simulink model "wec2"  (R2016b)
settings: Solver=ode4  StartTime=0  StopTime=350  FixedStep=0.005  MaxStep=0.005  RelTol=1e-3  EnableMultiTasking=on
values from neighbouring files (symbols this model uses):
  arAdaptiveLawData = 1/2*zModelSimple.zModelPto.arFreq.*     zModelSimple.zModelPto.arMagnitude./     cos(zModelSimple.zModelPto.arPhase*pi/180+pi/2)    [IMPACT_Control.m]
  arControllerRampGain = [0,0,1,1]    [IMPACT_Control.m]
  arControllerRampTime = [0 rStartRampTime rStartRampTime+rRampTimeLength 8000]    [IMPACT_Control.m]
  arEkfInitialisation = zeros(1,11)    [IMPACT_Control.m]
  arFrequency = zModelSimple.zModelPto.arFreq    [IMPACT_Control.m]
  arFrequencyRange = zModelSimple.zModelPto.arFreq    [IMPACT_Control.m]
  arImpedance = 1./zModelSimple.zModelPto.arMagnitude./zModelSimple.zModelPto.arFreq    [IMPACT_Control.m]
  iAdaptiveDamping = 0    [wec2_IMPACT_Project.m]    (also in IMPACT_Control.m = handles.iAdaptiveDamping; wec1_IMPACT_Project.m; wec3_IMPACT_Project.m; wec4IMPACT_Project.m)
  iControlType = 1    [wec2_IMPACT_Project.m]    (also in IMPACT_Control.m = handles.iControlType; wec1_IMPACT_Project.m; wec3_IMPACT_Project.m; wec4IMPACT_Project.m = 2)
  iPtoPositionConstraint = 1    [wec2_IMPACT_Project.m]    (also in IMPACT_Control.m = handles.iPtoPositionConstraint; wec1_IMPACT_Project.m = 0; wec3_IMPACT_Project.m; wec4IMPACT_Project.m)
  iSensorNoise = 0    [IMPACT_Control.m]
  m = m+1    (= 2)    [checkParamFile.m]
  rAccelerationGainPosLim = 4.5133e+06    (= 4513300)    [wec2AdditionalParams.m]    (also in wec1AdditionalParams.m = 9453000)
  rBalancingForce = -(rFloaterVolume*rDENSITY - rFloaterMass)*rGRAVITY    [IMPACT_Control.m]
  rBuoyancyGainPosLim = 7.4216    [wec2AdditionalParams.m]    (also in wec1AdditionalParams.m = 3135500)
  rCogFloater = -8.5    [wec2_IMPACT_Model.m]    (also in paramInitial.m = get( handles.edit_rCogFloater, 'String' ); wec1_IMPACT_Model.m = -18; wec3_IMPACT_Model.m = -0.7; wec3_IMPACT_Model2.m = -0.7)
  rDampingGainPosLim = 1.1575e+04    (= 11575)    [wec2AdditionalParams.m]    (also in wec1AdditionalParams.m = 203690)
  rDisplacementLimit = 10.000000    (= 10)    [wec2_IMPACT_Project.m]    (also in IMPACT_Control.m = getValue(handles.edit_displacementLimit); wec1_IMPACT_Project.m; wec3_IMPACT_Project.m = 3; wec4IMPACT_Project.m)
  rGainForAntiWIndUp = tfControllerDiscrete.rGain    [IMPACT_Control.m]
  rMaxForcePto = 1000000000000000.000000    (= 1e+15)    [wec2_IMPACT_Project.m]    (also in IMPACT_Control.m = getValue(handles.edit_maxForcePto); wec1_IMPACT_Project.m; wec3_IMPACT_Project.m = 1000000000; wec4IMPACT_Project.m = 300000000)
  rMinForcePto = -1000000000000000.000000    (= -1e+15)    [wec2_IMPACT_Project.m]    (also in IMPACT_Control.m = getValue(handles.edit_minForcePto); wec1_IMPACT_Project.m; wec3_IMPACT_Project.m = -1000000000; wec4IMPACT_Project.m = -300000000)
  rOutputSampleTime = 0.010000    (= 0.01)    [wec2_IMPACT_Project.m]    (also in IMPACT_Control.m = getValue(handles.edit_outputSampleTime); wec1_IMPACT_Project.m; wec3_IMPACT_Project.m; wec4IMPACT_Project.m)
  rPassiveDampingGain = -1948070.000000    (= -1948070)    [wec2_IMPACT_Project.m]    (also in IMPACT_Control.m = getValue(handles.edit_gainPLD); wec1_IMPACT_Project.m = -214018.1537; wec3_IMPACT_Project.m = -519390; wec4IMPACT_Project.m = -604830)
  rPositionLimitRatio = 10    [wec2AdditionalParams.m]    (also in wec1AdditionalParams.m)
  rUpperFrequencyLimit = EKFFloater.upperFreq    [IMPACT_Control.m]
  s = tf('s')    [wec2_IMPACT_Model.m]    (also in IMPACT_Control.m; wec1_IMPACT_Model.m; wec3_IMPACT_Model.m; wec3_IMPACT_Model2.m)
  simu = simulationClass()    [wecSimInputFile.m]
  Z = magPhaseToComplex(zModelTf)    [IMPACT_Control.m]
undefined symbols (not defined in the file or in its folder): arControllerDiscreteDen, arControllerDiscreteNum, arExcForceFloaterDen, arExcForceFloaterNum, body, N, pto, rAccelerationGainFloater, rBuoyancyGainFloater, rDampingGainFloater, X, Y
libraries: nesl_utility x9, sm_lib x5, simulink x3, WECSim_Lib x2

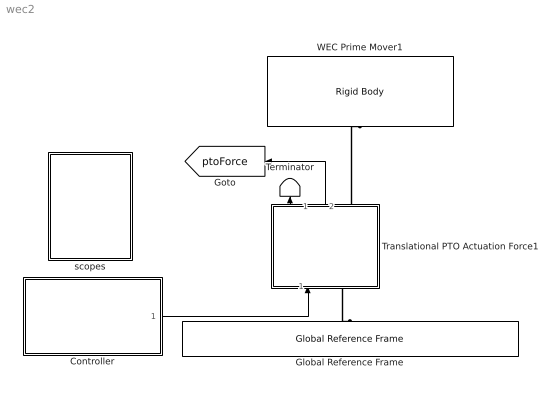
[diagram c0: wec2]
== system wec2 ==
  Controller : Subsystem
  Global Reference Frame : WECSim_Lib/Frames/Global Reference Frame  waves=waves  simu=simu
  Terminator : Terminator
  Translational PTO Actuation Force1 : Subsystem  AncestorBlock=WECSim_Lib/PTOs/Translational PTO Actuation Force
  WEC Prime Mover1 : WECSim_Lib/Body Elements/Rigid Body  body=body(1)
  scopes : Subsystem
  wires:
  Translational PTO Actuation Force1/2(ptoForce) -> [ptoForce]
  Controller/1(forceDemand) -> Translational PTO Actuation Force1/1(Force)
  Translational PTO Actuation Force1/1(Response) -> Terminator/1
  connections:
  Translational PTO Actuation Force1/LConn1 -- Global Reference Frame/RConn1
  Translational PTO Actuation Force1/RConn1 -- WEC Prime Mover1/RConn1

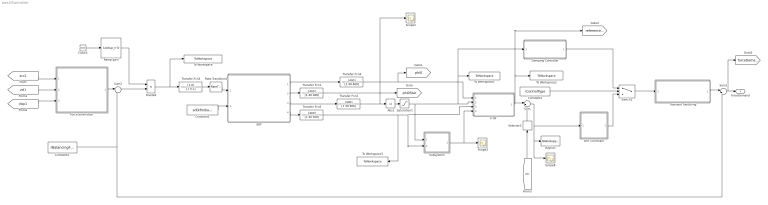
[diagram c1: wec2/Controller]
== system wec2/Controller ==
  Abs1 : Abs
  Clock3 : Clock
  Constant1 : Constant  Value=arEkfInitialisation
  Constant2 : Constant  Value=iControlType
  Constant5 : Constant  Value=rBalancingForce
  Damping Controller : Subsystem
  Divide4 : Product  Inputs=**
  EKF : MATLAB Function  TreatAsAtomicUnit=on
  "Force estimation " : Subsystem
  OVT Controller : Subsystem
  Ramp gain : Lookup_n-D  NumberOfTableDimensions=1  BreakpointsForDimension1=[0 5 10 8000]  Table=[0 0 1 1]  InternalRulePriority=Speed  RndMeth=Simplest
  Rate Transition1 : RateTransition  OutPortSampleTimeMultiple=0.01  OutPortSampleTime=0.01
  Saturation1 : Saturate  UpperLimit=rUpperFrequencyLimit  LowerLimit=0  LinearizeAsGain=off
  Scope2 : Scope
  Scope3 : Scope
  Scope8 : Scope
  Selector2 : Selector  InputPortWidth=6  IndexOptions=Index vector (dialog)  Indices=3  OutputSizes=1
  Subsystem : Subsystem
  Sum : Sum  Inputs=|+-
  Sum1 : Sum  Inputs=|++
  Sum2 : Sum  Inputs=|++
  Switch1 : Switch  Threshold=2
  To Workspace : ToWorkspace  VariableName=arEstimatedExcitationForce  SampleTime=rOutputSampleTime
  To Workspace1 : ToWorkspace  VariableName=arEkfFrequency  SampleTime=rOutputSampleTime
  To Workspace2 : ToWorkspace  VariableName=arReferenceVelocity  SampleTime=rOutputSampleTime
  To Workspace3 : ToWorkspace  VariableName=arEkfAmplitude  SampleTime=rOutputSampleTime
  Transfer Fcn{1..2,4..5} (4 alike) : TransferFcn  Numerator=[400]  Denominator=[1 40 400]
  Transfer Fcn3 : TransferFcn  Numerator=[1 0]  Denominator=[1 0.1]
  Transient Switching : Subsystem
  "V ref " : Subsystem
  output1 : ToWorkspace  VariableName=arError  SampleTime=rOutputSampleTime
  forceDemand : Outport
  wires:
  Damping Controller/1(forceDemand) -> Switch1/1
  Sum/1 -> output1/1, Scope8/1, OVT Controller/1(error)
  Selector2/1 -> Sum/2
  "V ref "/1(referenceVelocity) -> Sum/1, To Workspace2/1, [referenceVelocity]
  [vel1] -> Selector2/1
  Constant2/1 -> Switch1/2
  OVT Controller/1(forceDemand) -> Switch1/3
  Saturation1/1 -> Subsystem/1(frequency), Damping Controller/1(ekfFrequency), To Workspace1/1, "V ref "/2(ekfFrequency)
  [acc1] -> "Force estimation "/1(Acceleration)
  [vel1] -> "Force estimation "/2(Velocity)
  [disp1] -> "Force estimation "/3(Position)
  Abs1/1 -> Saturation1/1
  "Force estimation "/1(estimatedExcitationForce) -> Sum2/1
  Sum1/1 -> [forceDemand], forceDemand/1
  Constant1/1 -> EKF/2(arEkfInitialisation)
  Constant5/1 -> Sum1/2, Sum2/2
  Switch1/1 -> Transient Switching/1(forceDemandIn)
  Transient Switching/1(forceDemandOut) -> Sum1/1
  Rate Transition1/1 -> EKF/1(rEstimatedExcitationForce)
  Sum2/1 -> Divide4/2
  EKF/4(rAmplitudeOutput) -> Transfer Fcn5/1
  EKF/3(rFrequencyOutput) -> Transfer Fcn2/1
  EKF/1(rPhi0Output) -> Transfer Fcn4/1
  EKF/2(rPhi0StarOutput) -> Transfer Fcn1/1
  Transfer Fcn5/1 -> Subsystem/2(excitationForce), "V ref "/3(ekfAmplitude), To Workspace3/1
  Transfer Fcn2/1 -> Abs1/1, Scope2/1
  Transfer Fcn1/1 -> [phi0Star]
  Transfer Fcn4/1 -> [phi0], "V ref "/1(phiOut)
  Subsystem/1(displacementLimit) -> Scope3/1, "V ref "/4(displacementLimit)
  Clock3/1 -> Ramp gain/1
  Ramp gain/1 -> Divide4/1
  Divide4/1 -> To Workspace/1, Transfer Fcn3/1
  Transfer Fcn3/1 -> Rate Transition1/1

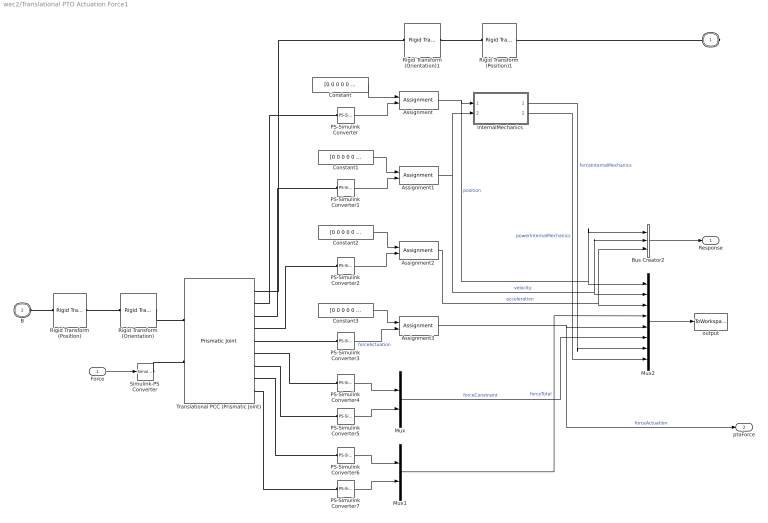
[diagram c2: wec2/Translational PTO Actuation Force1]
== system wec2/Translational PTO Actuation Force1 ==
  Force : Inport
  Assignment{,1..3} (4 alike) : Assignment  IndexOptions=Index vector (dialog)  Indices=3  OutputSizes=1
  Bus Creator2 : BusCreator  Inputs=3
  Constant{,1..3} (4 alike) : Constant  Value=[0 0 0 0 0 0]
  InternalMechanics : Subsystem
  Mux : Mux  Inputs=2
  Mux1 : Mux  Inputs=2
  Mux2 : Mux  Inputs=8
  PS-Simulink Converter{,1..7} (8 alike) : nesl_utility/PS-Simulink Converter  PhysicalDomain=network_engine_domain  SubClassName=ps_output  LeftPortType=input  RightPortType=output  PseudoPeriodic=off  Frequencies=[]  Unit=1  AffineConversion=off
  Rigid Transform (Position) : sm_lib/Frames and Transforms/Rigid Transform  TranslationMethod=Cartesian  TranslationStandardOffset=0  TranslationLengthUnit=m  TranslationStandardAxis=+Z  TranslationCartesianOffset=pto.initDisp.initLinDisp + pto.loc  TranslationROffset=0  TranslationROffsetUnits=m  TranslationZOffset=0  TranslationZOffsetUnits=m  TranslationThetaOffset=0  TranslationThetaOffsetUnits=deg  RotationMethod=None  RotationAngleUnits=rad  RotationStandardAxis=+Y  RotationAngle=0  RotationArbitraryAxis=[0 1 0]  FollAlignAxisA=+X  BaseAlignAxisA=+Y  FollAlignAxisB=+Y  BaseAlignAxisB=+Z  RotationSequenceAxes=FollowerAxes  RotationSequence=XYX  RotationSequenceAngles=[0 0 0]  RotationSequenceAnglesUnits=deg  RotationMatrix=[1 0 0; 0 1 0; 0 0 1]
  Rigid Transform (Position)1 : sm_lib/Frames and Transforms/Rigid Transform  TranslationMethod=Cartesian  TranslationStandardOffset=0  TranslationLengthUnit=m  TranslationStandardAxis=+Z  TranslationCartesianOffset=pto.initDisp.initLinDisp + pto.loc  TranslationROffset=0  TranslationROffsetUnits=m  TranslationZOffset=0  TranslationZOffsetUnits=m  TranslationThetaOffset=0  TranslationThetaOffsetUnits=deg  RotationMethod=None  RotationAngleUnits=rad  RotationStandardAxis=+Y  RotationAngle=0  RotationArbitraryAxis=[0 1 0]  FollAlignAxisA=+X  BaseAlignAxisA=+Y  FollAlignAxisB=+Y  BaseAlignAxisB=+Z  RotationSequenceAxes=FollowerAxes  RotationSequence=XYX  RotationSequenceAngles=[0 0 0]  RotationSequenceAnglesUnits=deg  RotationMatrix=[1 0 0; 0 1 0; 0 0 1]
  Rigid Transform (Orientation) : sm_lib/Frames and Transforms/Rigid Transform  TranslationMethod=None  TranslationStandardOffset=0  TranslationLengthUnit=m  TranslationStandardAxis=+Z  TranslationCartesianOffset=0  TranslationROffset=0  TranslationROffsetUnits=m  TranslationZOffset=0  TranslationZOffsetUnits=m  TranslationThetaOffset=0  TranslationThetaOffsetUnits=deg  RotationMethod=RotationMatrix  RotationAngleUnits=rad  RotationStandardAxis=+Y  RotationAngle=0  RotationArbitraryAxis=[0 1 0]  FollAlignAxisA=+X  BaseAlignAxisA=+Y  FollAlignAxisB=+Y  BaseAlignAxisB=+Z  RotationSequenceAxes=FollowerAxes  RotationSequence=XYX  RotationSequenceAngles=[0 0 0]  RotationSequenceAnglesUnits=deg  RotationMatrix=pto.orientation.rotationMatrix
  Rigid Transform (Orientation)1 : sm_lib/Frames and Transforms/Rigid Transform  TranslationMethod=None  TranslationStandardOffset=0  TranslationLengthUnit=m  TranslationStandardAxis=+Z  TranslationCartesianOffset=0  TranslationROffset=0  TranslationROffsetUnits=m  TranslationZOffset=0  TranslationZOffsetUnits=m  TranslationThetaOffset=0  TranslationThetaOffsetUnits=deg  RotationMethod=RotationMatrix  RotationAngleUnits=rad  RotationStandardAxis=+Y  RotationAngle=0  RotationArbitraryAxis=[0 1 0]  FollAlignAxisA=+X  BaseAlignAxisA=+Y  FollAlignAxisB=+Y  BaseAlignAxisB=+Z  RotationSequenceAxes=FollowerAxes  RotationSequence=XYX  RotationSequenceAngles=[0 0 0]  RotationSequenceAnglesUnits=deg  RotationMatrix=pto.orientation.rotationMatrix
  Simulink-PS Converter : nesl_utility/Simulink-PS Converter  PhysicalDomain=network_engine_domain  SubClassName=ps_input  LeftPortType=input  RightPortType=output  PseudoPeriodic=off  Frequencies=[]  NoiseDistribution=none  NoiseParameters=[]  Unit=1  AffineConversion=off  InputFiltering=off  SimscapeFilterOrder=1  InputFilterTimeConstant=0.001  UdotUserProvided=1
  Translational PCC (Prismatic Joint) : sm_lib/Joints/Prismatic Joint  SenseConstraintForce=on  SenseConstraintForceX=off  SenseConstraintForceY=off  SenseConstraintForceZ=off  SenseConstraintTorque=on  SenseConstraintTorqueX=off  SenseConstraintTorqueY=off  SenseConstraintTorqueZ=off  SenseTotalForce=on  SenseTotalForceX=off  SenseTotalForceY=off  SenseTotalForceZ=off  SenseTotalTorque=on  SenseTotalTorqueX=off  SenseTotalTorqueY=off  SenseTotalTorqueZ=off  CompositeWrenchDir=BaseOnFollower  CompositeWrenchFrame=BaseFrame  EquilibriumPosition=0  EquilibriumPositionUnits=m  SpringStiffness=pto.k  SpringStiffnessUnits=N/m  DampingCoefficient=pto.c  DampingCoefficientUnits=N/(m/s)  TorqueActuationMode=InputTorque  MotionActuationMode=ComputedMotion  SensePosition=on  SenseVelocity=on  SenseAcceleration=on  SenseTorqueForce=on  PositionTargetSpecify=off  PositionTargetPriority=High  PositionTargetValue=0  PositionTargetValueUnits=m  VelocityTargetSpecify=off  VelocityTargetPriority=High  VelocityTargetValue=0  VelocityTargetValueUnits=m/s
  output : ToWorkspace  VariableName=pto1_out  SaveFormat=Structure With Time  SampleTime=-1
  F : PMIOPort  Port=1  Side=Right
  B : PMIOPort  Port=2  Side=Left
  Response : Outport
  ptoForce : Outport  Port=2
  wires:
  Bus Creator2/1 -> Response/1
  Assignment/1 -> Mux2/1, Bus Creator2/1, InternalMechanics/1(Position)  "position"
  Assignment1/1 -> Mux2/2, Bus Creator2/2, InternalMechanics/2(Velocity)  "velocity"
  Assignment2/1 -> Mux2/3, Bus Creator2/3  "acceleration"
  Force/1 -> Simulink-PS Converter/1
  Mux2/1 -> output/1
  Mux/1 -> Mux2/6  "forceConstraint"
  Mux1/1 -> Mux2/4  "forceTotal"
  PS-Simulink Converter4/1 -> Mux/1
  PS-Simulink Converter5/1 -> Mux/2
  PS-Simulink Converter6/1 -> Mux1/1
  PS-Simulink Converter7/1 -> Mux1/2
  Assignment3/1 -> ptoForce/1, Mux2/5  "forceActuation"
  Constant/1 -> Assignment/1
  PS-Simulink Converter/1 -> Assignment/2
  Constant1/1 -> Assignment1/1
  PS-Simulink Converter1/1 -> Assignment1/2
  Constant2/1 -> Assignment2/1
  PS-Simulink Converter2/1 -> Assignment2/2
  InternalMechanics/1(Force) -> Mux2/7  "forceInternalMechanics"
  InternalMechanics/2(Power) -> Mux2/8  "powerInternalMechanics"
  Constant3/1 -> Assignment3/1
  PS-Simulink Converter3/1 -> Assignment3/2  "forceActuation"
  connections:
  Rigid Transform (Position)/RConn1 -- Rigid Transform (Orientation)/LConn1
  Rigid Transform (Position)1/RConn1 -- Rigid Transform (Orientation)1/LConn1
  Simulink-PS Converter/RConn1 -- Translational PCC (Prismatic Joint)/LConn2
  Rigid Transform (Orientation)/RConn1 -- Translational PCC (Prismatic Joint)/LConn1
  Rigid Transform (Position)/LConn1 -- B/RConn1
  Translational PCC (Prismatic Joint)/RConn5 -- PS-Simulink Converter3/LConn1
  Translational PCC (Prismatic Joint)/RConn9 -- PS-Simulink Converter7/LConn1
  Rigid Transform (Orientation)1/RConn1 -- Translational PCC (Prismatic Joint)/RConn1
  Translational PCC (Prismatic Joint)/RConn4 -- PS-Simulink Converter2/LConn1
  Translational PCC (Prismatic Joint)/RConn7 -- PS-Simulink Converter5/LConn1
  Translational PCC (Prismatic Joint)/RConn3 -- PS-Simulink Converter1/LConn1
  Rigid Transform (Position)1/LConn1 -- F/RConn1
  Translational PCC (Prismatic Joint)/RConn8 -- PS-Simulink Converter6/LConn1
  Translational PCC (Prismatic Joint)/RConn2 -- PS-Simulink Converter/LConn1
  Translational PCC (Prismatic Joint)/RConn6 -- PS-Simulink Converter4/LConn1

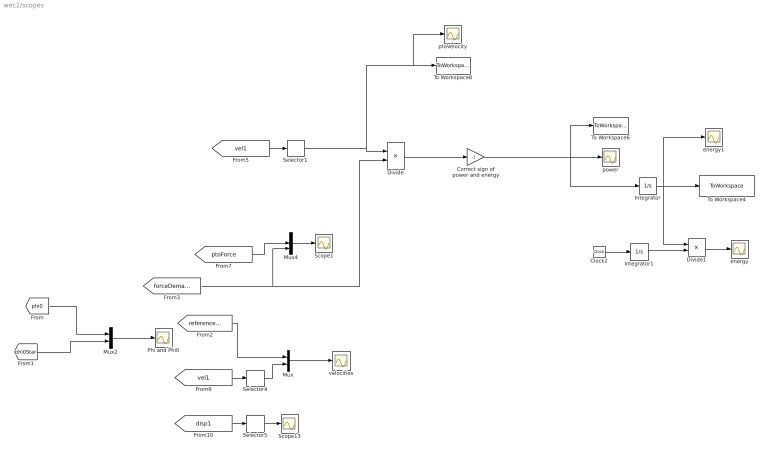
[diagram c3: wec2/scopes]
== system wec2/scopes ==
  Clock2 : Clock
  Correct sign of power and energy : Gain  Gain=-1
  Divide : Product  Inputs=**
  Divide1 : Product  Inputs=*/
  Integrator : Integrator
  Integrator1 : Integrator
  Mux : Mux  Inputs=2
  Mux2 : Mux  Inputs=2
  Mux4 : Mux  Inputs=3
  Phi and Phi0 : Scope
  Scope1 : Scope
  Scope13 : Scope
  Selector1 : Selector  InputPortWidth=6  IndexOptions=Index vector (dialog)  Indices=3  OutputSizes=1
  Selector4 : Selector  InputPortWidth=6  IndexOptions=Index vector (dialog)  Indices=3  OutputSizes=1
  Selector5 : Selector  InputPortWidth=6  IndexOptions=Index vector (dialog)  Indices=3  OutputSizes=1
  To Workspace4 : ToWorkspace  VariableName=arWecEnergy  SampleTime=rOutputSampleTime
  To Workspace6 : ToWorkspace  VariableName=arWecPower  SampleTime=rOutputSampleTime
  To Workspace8 : ToWorkspace  VariableName=arPtoVelocity  SampleTime=rOutputSampleTime
  energy : Scope
  energy1 : Scope
  power : Scope
  ptoVelocity : Scope
  velocities : Scope
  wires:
  [vel1] -> Selector4/1
  Mux/1 -> velocities/1
  Selector5/1 -> Scope13/1
  [phi0] -> Mux2/1
  Mux2/1 -> Phi and Phi0/1
  Mux4/1 -> Scope1/1
  [ptoForce] -> Mux4/2
  Selector4/1 -> Mux/2
  [disp1] -> Selector5/1
  [referenceVelocity] -> Mux/1
  [forceDemand] -> Divide/2, Mux4/3
  Clock2/1 -> Integrator1/1
  Divide1/1 -> energy/1
  Integrator1/1 -> Divide1/2
  Integrator/1 -> energy1/1, To Workspace4/1, Divide1/1
  Divide/1 -> Correct sign of power and energy/1
  Selector1/1 -> Divide/1, ptoVelocity/1, To Workspace8/1
  [vel1] -> Selector1/1
  [phi0Star] -> Mux2/2
  Correct sign of power and energy/1 -> Integrator/1, To Workspace6/1, power/1

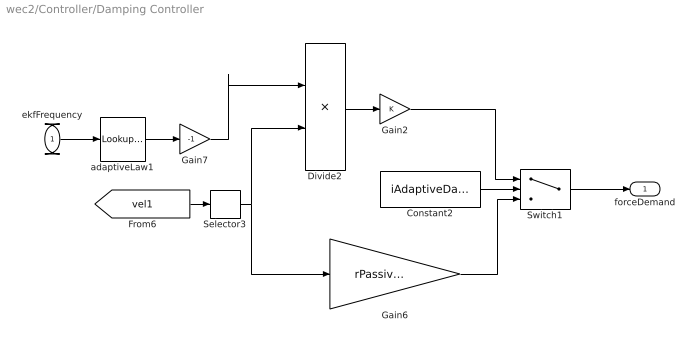
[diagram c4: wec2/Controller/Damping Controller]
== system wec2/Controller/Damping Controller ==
  ekfFrequency : Inport
  Constant2 : Constant  Value=iAdaptiveDamping
  Divide2 : Product  Inputs=**
  Gain2 : Gain
  Gain6 : Gain  Gain=rPassiveDampingGain
  Gain7 : Gain  Gain=-1
  Selector3 : Selector  InputPortWidth=6  IndexOptions=Index vector (dialog)  Indices=3  OutputSizes=1
  Switch1 : Switch  Criteria=u2 > Threshold
  adaptiveLaw1 : Lookup_n-D  NumberOfTableDimensions=1  BreakpointsForDimension1=arFrequency  Table=arImpedance  InternalRulePriority=Speed  RndMeth=Simplest
  forceDemand : Outport
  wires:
  Gain2/1 -> Switch1/1
  ekfFrequency/1 -> adaptiveLaw1/1
  adaptiveLaw1/1 -> Gain7/1
  Constant2/1 -> Switch1/2
  Switch1/1 -> forceDemand/1
  Gain7/1 -> Divide2/1
  Selector3/1 -> Divide2/2, Gain6/1
  [vel1] -> Selector3/1
  Divide2/1 -> Gain2/1
  Gain6/1 -> Switch1/3

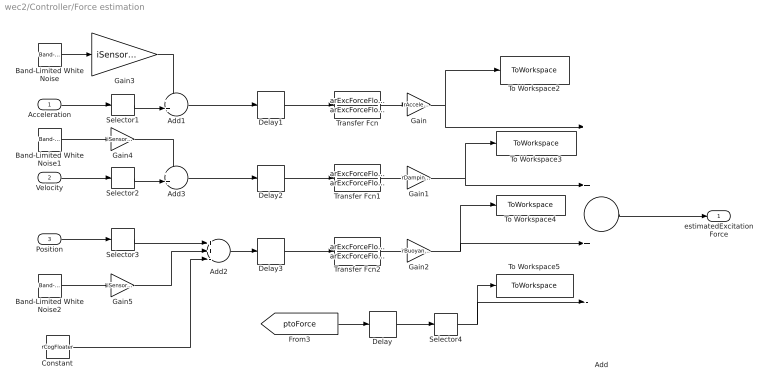
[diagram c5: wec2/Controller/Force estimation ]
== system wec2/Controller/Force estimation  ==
  Acceleration : Inport
  Velocity : Inport  Port=2
  Position : Inport  Port=3
  Add : Sum  Inputs=+++-
  Add1 : Sum  Inputs=++|
  Add2 : Sum  Inputs=++-
  Add3 : Sum  Inputs=++|
  Band-Limited White Noise : simulink/Sources/Band-Limited White Noise  Cov=rAccNoisePower  Ts=simu.dt  seed=[23341]
  Band-Limited White Noise1 : simulink/Sources/Band-Limited White Noise  Cov=rVelNoisePower  Ts=simu.dt  seed=[23341]
  Band-Limited White Noise2 : simulink/Sources/Band-Limited White Noise  Cov=rPosNoisePower  Ts=simu.dt  seed=[23341]
  Constant : Constant  Value=rCogFloater
  Delay{,1..3} (4 alike) : Delay  DelayLength=1  SampleTime=0.01
  Gain : Gain  Gain=rAccelerationGainFloater
  Gain1 : Gain  Gain=rDampingGainFloater
  Gain2 : Gain  Gain=rBuoyancyGainFloater
  Gain3 : Gain  Gain=iSensorNoise
  Gain4 : Gain  Gain=iSensorNoise
  Gain5 : Gain  Gain=iSensorNoise
  Selector{1..4} (4 alike) : Selector  InputPortWidth=6  IndexOptions=Index vector (dialog)  Indices=3  OutputSizes=1
  To Workspace2 : ToWorkspace  VariableName=arAccelerationComponent  SampleTime=rOutputSampleTime
  To Workspace3 : ToWorkspace  VariableName=arVelocityComponent  SampleTime=rOutputSampleTime
  To Workspace4 : ToWorkspace  VariableName=arPositionComponent  SampleTime=rOutputSampleTime
  To Workspace5 : ToWorkspace  VariableName=arPtoForceMeasurement  SampleTime=rOutputSampleTime
  Transfer Fcn : TransferFcn  Numerator=arExcForceFloaterNum  Denominator=arExcForceFloaterDen
  Transfer Fcn1 : TransferFcn  Numerator=arExcForceFloaterNum  Denominator=arExcForceFloaterDen
  Transfer Fcn2 : TransferFcn  Numerator=arExcForceFloaterNum  Denominator=arExcForceFloaterDen
  estimatedExcitationForce : Outport
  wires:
  Selector1/1 -> Add1/2
  Band-Limited White Noise/1 -> Gain3/1
  Acceleration/1 -> Selector1/1
  Gain5/1 -> Add2/2
  Add2/1 -> Delay3/1
  Position/1 -> Selector3/1
  Add/1 -> estimatedExcitationForce/1
  [ptoForce] -> Delay/1
  Gain/1 -> Add/1, To Workspace2/1
  Constant/1 -> Add2/3
  Gain4/1 -> Add3/1
  Velocity/1 -> Selector2/1
  Gain3/1 -> Add1/1
  Selector2/1 -> Add3/2
  Add1/1 -> Delay1/1
  Selector3/1 -> Add2/1
  Band-Limited White Noise1/1 -> Gain4/1
  Band-Limited White Noise2/1 -> Gain5/1
  Selector4/1 -> Add/4, To Workspace5/1
  Delay/1 -> Selector4/1
  Gain1/1 -> To Workspace3/1, Add/2
  Add3/1 -> Delay2/1
  Delay1/1 -> Transfer Fcn/1
  Delay2/1 -> Transfer Fcn1/1
  Transfer Fcn1/1 -> Gain1/1
  Transfer Fcn/1 -> Gain/1
  Delay3/1 -> Transfer Fcn2/1
  Transfer Fcn2/1 -> Gain2/1
  Gain2/1 -> To Workspace4/1, Add/3

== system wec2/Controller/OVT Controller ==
  error : Inport
  Anti wind-up controller : Subsystem
  forceDemand : Outport
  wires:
  error/1 -> Anti wind-up controller/1(error)
  Anti wind-up controller/1(Out1) -> forceDemand/1

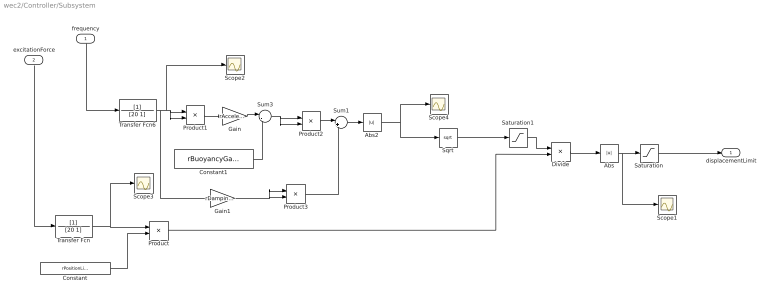
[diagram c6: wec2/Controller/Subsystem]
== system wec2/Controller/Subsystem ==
  frequency : Inport
  excitationForce : Inport  Port=2
  Abs : Abs
  Abs2 : Abs
  Constant : Constant  Value=rPositionLimitRatio
  Constant1 : Constant  Value=rBuoyancyGainPosLim
  Divide : Product  Inputs=/*
  Gain : Gain  Gain=rAccelerationGainPosLim
  Gain1 : Gain  Gain=rDampingGainPosLim
  Product{,1..3} (4 alike) : Product
  Saturation : Saturate  UpperLimit=10  LowerLimit=0
  Saturation1 : Saturate  UpperLimit=inf  LowerLimit=0.0001
  Scope{1..4} (4 alike) : Scope
  Sqrt : Sqrt
  Sum1 : Sum  Inputs=|++
  Sum3 : Sum  Inputs=|-+
  Transfer Fcn : TransferFcn  Denominator=[20 1]
  Transfer Fcn6 : TransferFcn  Denominator=[20 1]
  displacementLimit : Outport
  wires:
  Product1/1 -> Gain/1
  Gain/1 -> Sum3/1
  Transfer Fcn6/1 -> Gain1/1, Scope2/1, Product1/2, Product1/1
  Constant1/1 -> Sum3/2
  Product/1 -> Divide/2
  Constant/1 -> Product/2
  Transfer Fcn/1 -> Scope3/1, Product/1
  frequency/1 -> Transfer Fcn6/1
  excitationForce/1 -> Transfer Fcn/1
  Divide/1 -> Abs/1
  Sum3/1 -> Product2/1, Product2/2
  Abs/1 -> Scope1/1, Saturation/1
  Saturation/1 -> displacementLimit/1
  Saturation1/1 -> Divide/1
  Abs2/1 -> Scope4/1, Sqrt/1
  Product2/1 -> Sum1/1
  Gain1/1 -> Product3/1, Product3/2
  Product3/1 -> Sum1/2
  Sum1/1 -> Abs2/1
  Sqrt/1 -> Saturation1/1

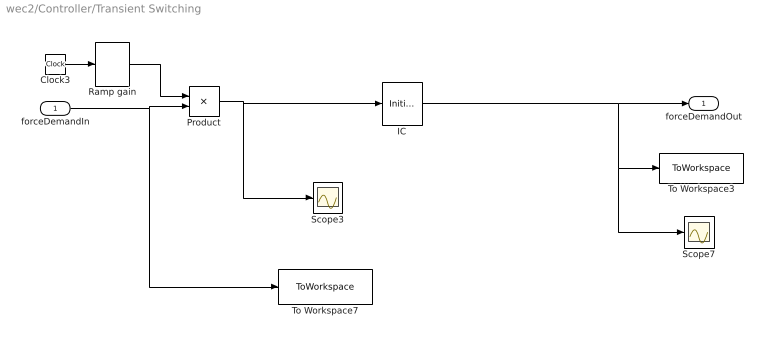
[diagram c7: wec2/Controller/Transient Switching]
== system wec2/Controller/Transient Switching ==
  forceDemandIn : Inport
  Clock3 : Clock
  IC : InitialCondition  Value=0
  Product : Product
  Ramp gain : Lookup_n-D  NumberOfTableDimensions=1  BreakpointsForDimension1=arControllerRampTime  Table=arControllerRampGain  InternalRulePriority=Speed  RndMeth=Simplest
  Scope3 : Scope
  Scope7 : Scope
  To Workspace3 : ToWorkspace  VariableName=arForceDemand  SampleTime=rOutputSampleTime
  To Workspace7 : ToWorkspace  VariableName=arForceDemandIn  SampleTime=rOutputSampleTime
  forceDemandOut : Outport
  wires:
  Clock3/1 -> Ramp gain/1
  forceDemandIn/1 -> Product/2, To Workspace7/1
  Ramp gain/1 -> Product/1
  Product/1 -> IC/1, Scope3/1
  IC/1 -> To Workspace3/1, Scope7/1, forceDemandOut/1

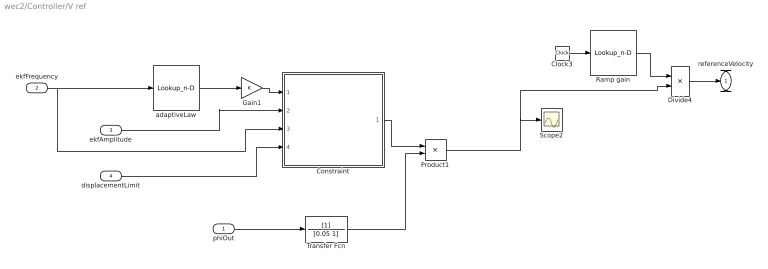
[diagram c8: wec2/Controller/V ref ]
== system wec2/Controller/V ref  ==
  phiOut : Inport
  ekfFrequency : Inport  Port=2
  ekfAmplitude : Inport  Port=3
  displacementLimit : Inport  Port=4
  Clock3 : Clock
  Constraint : Subsystem
  Divide4 : Product  Inputs=**
  Gain1 : Gain
  Product1 : Product
  Ramp gain : Lookup_n-D  NumberOfTableDimensions=1  BreakpointsForDimension1=arControllerRampTime  Table=arControllerRampGain  InternalRulePriority=Speed  RndMeth=Simplest
  Scope2 : Scope
  Transfer Fcn : TransferFcn  Denominator=[0.05 1]
  adaptiveLaw : Lookup_n-D  NumberOfTableDimensions=1  BreakpointsForDimension1=arFrequencyRange  Table=arAdaptiveLawData  InternalRulePriority=Speed  RndMeth=Simplest
  referenceVelocity : Outport
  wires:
  Constraint/1(referenceVelocity) -> Product1/1
  Ramp gain/1 -> Divide4/1
  Clock3/1 -> Ramp gain/1
  Gain1/1 -> Constraint/1(1/2B)
  adaptiveLaw/1 -> Gain1/1
  Divide4/1 -> referenceVelocity/1
  ekfFrequency/1 -> Constraint/3(ekfFrequency), adaptiveLaw/1
  phiOut/1 -> Transfer Fcn/1
  ekfAmplitude/1 -> Constraint/2(Amp)
  Product1/1 -> Divide4/2, Scope2/1
  Transfer Fcn/1 -> Product1/2
  displacementLimit/1 -> Constraint/4(displacementLimit)

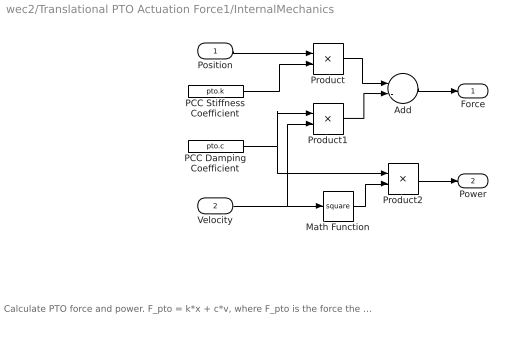
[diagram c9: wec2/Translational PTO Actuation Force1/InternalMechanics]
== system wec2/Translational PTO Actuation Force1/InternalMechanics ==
  note: Calculate PTO force and power. F_pto = k*x + c*v, where F_pto is the force the PTO applies to the body (at the PTO location), x and v are the joint position and velocity. The power extracted is P = c * v^2
  Position : Inport
  Velocity : Inport  Port=2
  Add : Sum  Inputs=--
  Math Function : Math  Operator=square
  PCC Damping Coefficient : Constant  Value=pto.c
  PCC Stiffness Coefficient : Constant  Value=pto.k
  Product : Product  Inputs=**
  Product1 : Product  Inputs=**
  Product2 : Product  Inputs=**
  Force : Outport
  Power : Outport  Port=2
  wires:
  PCC Damping Coefficient/1 -> Product2/1, Product1/1
  Product2/1 -> Power/1
  Velocity/1 -> Math Function/1, Product1/2
  PCC Stiffness Coefficient/1 -> Product/2
  Position/1 -> Product/1
  Add/1 -> Force/1
  Math Function/1 -> Product2/2
  Product/1 -> Add/1
  Product1/1 -> Add/2

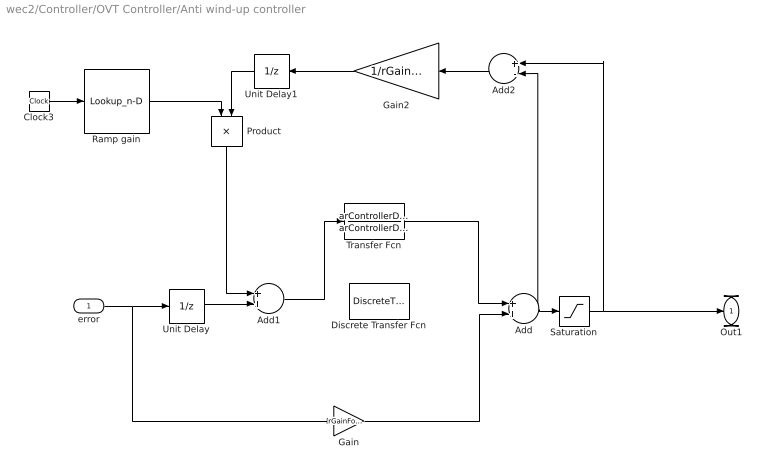
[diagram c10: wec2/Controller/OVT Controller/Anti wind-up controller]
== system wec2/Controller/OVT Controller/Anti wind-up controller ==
  error : Inport
  Add : Sum
  Add1 : Sum
  Add2 : Sum  Inputs=+-
  Clock3 : Clock
  Discrete Transfer Fcn : DiscreteTransferFcn  Numerator=arControllerDiscreteNum  Denominator=arControllerDiscreteDen
  Gain : Gain  Gain=rGainForAntiWIndUp
  Gain2 : Gain  Gain=1/rGainForAntiWIndUp
  Product : Product
  Ramp gain : Lookup_n-D  NumberOfTableDimensions=1  BreakpointsForDimension1=arControllerRampTime  Table=arControllerRampGain  InternalRulePriority=Speed  RndMeth=Simplest
  Saturation : Saturate  UpperLimit=rMaxForcePto  LowerLimit=rMinForcePto
  Transfer Fcn : TransferFcn  Numerator=arControllerDiscreteNum  Denominator=arControllerDiscreteDen
  Unit Delay : UnitDelay  SampleTime=0.01
  Unit Delay1 : UnitDelay  SampleTime=0.01
  Out1 : Outport
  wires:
  Add/1 -> Saturation/1, Add2/2
  Gain/1 -> Add/2
  Unit Delay/1 -> Add1/2
  Gain2/1 -> Unit Delay1/1
  error/1 -> Gain/1, Unit Delay/1
  Add2/1 -> Gain2/1
  Add1/1 -> Transfer Fcn/1
  Discrete Transfer Fcn/1 -> ?
  Clock3/1 -> Ramp gain/1
  Ramp gain/1 -> Product/1
  Product/1 -> Add1/1
  Unit Delay1/1 -> Product/2
  Saturation/1 -> Add2/1, Out1/1
  Transfer Fcn/1 -> Add/1

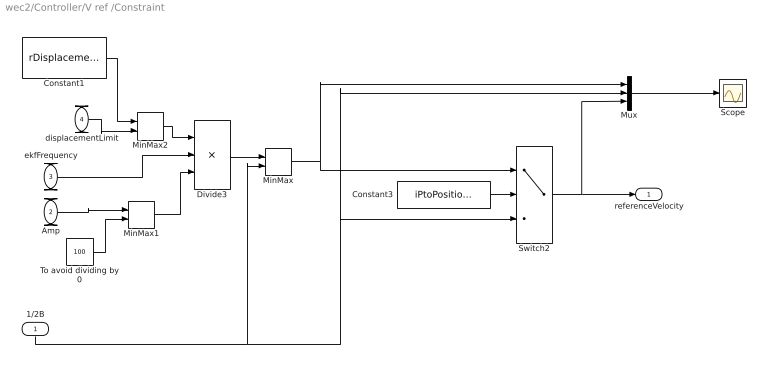
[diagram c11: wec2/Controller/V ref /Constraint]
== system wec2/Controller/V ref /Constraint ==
  1/2B : Inport
  Amp : Inport  Port=2
  ekfFrequency : Inport  Port=3
  displacementLimit : Inport  Port=4
  Constant1 : Constant  Value=rDisplacementLimit
  Constant3 : Constant  Value=iPtoPositionConstraint
  Divide3 : Product  Inputs=**/
  MinMax : MinMax  Inputs=2
  MinMax1 : MinMax  Function=max  Inputs=2
  MinMax2 : MinMax  Inputs=2
  Mux : Mux  Inputs=3
  Scope : Scope
  Switch2 : Switch  Criteria=u2 > Threshold
  To avoid dividing by 0 : Constant  Value=100
  referenceVelocity : Outport
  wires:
  MinMax/1 -> Mux/1, Switch2/1
  ekfFrequency/1 -> Divide3/2
  MinMax2/1 -> Divide3/1
  MinMax1/1 -> Divide3/3
  Divide3/1 -> MinMax/1
  To avoid dividing by 0/1 -> MinMax1/2
  Amp/1 -> MinMax1/1
  Constant3/1 -> Switch2/2
  Switch2/1 -> Mux/3, referenceVelocity/1
  Mux/1 -> Scope/1
  1/2B/1 -> MinMax/2, Switch2/3, Mux/2
  Constant1/1 -> MinMax2/1
  displacementLimit/1 -> MinMax2/2

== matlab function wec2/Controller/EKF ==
function [rPhi0Output,rPhi0StarOutput,rFrequencyOutput, rAmplitudeOutput]...
    = kalmanFilter(rEstimatedExcitationForce,arEkfInitialisation)
%%%%%%%%%%%%%%%%%%%%%%%%%%%%%%%%%%%%%%%%%%%%%%%%%%%%%%%%%%%%%%%%%%%%%%%%%
%%%                     Extended Kalman Filter                        %%%

%-----------------------------
% State equations
% X[n+1] = A*X[n] + B*U[n] + v
% Output equation
% Y[n] = C*X[n] + e
%-----------------------------
% n = Nº States
% m = Nº of inputs
% p = Nº of outputs
%
% See the IMPACT Deliverable 4 report for more detail on derivation of the
% Extended Kalman Filter
%
%%%%%%%%%%%%%%%%%%%%%%%%%%%%%%%%%%%%%%%%%%%%%%%%%%%%%%%%%%%%%%%%%%%%%%%%%

% Matrices of the system: A, B, C

persistent A B C P_k_k R1 R2 X_k_k bInit rFrequency rTimeStep rPhi0 rPhi0Star 

% On the first step bInit is empty and so the initialisation can run

if isempty(bInit)
    
    bInit = 1;
    rFrequency = arEkfInitialisation(1);%0.5;
    rPhi0 = arEkfInitialisation(2);%1e5;
    rPhi0Star = arEkfInitialisation(3);%0;
    rTimeStep = arEkfInitialisation(4);
    
    A = zeros(3);
    A(1,:) = [cos(rFrequency*rTimeStep), sin(rFrequency*rTimeStep),...
        (-sin(rFrequency*rTimeStep)*rPhi0+cos(rFrequency*rTimeStep)*rPhi0Star)*rTimeStep];
    A(2,:) = [-sin(rFrequency*rTimeStep), cos(rFrequency*rTimeStep),...
        (-cos(rFrequency*rTimeStep)*rPhi0-sin(rFrequency*rTimeStep)*rPhi0Star)*rTimeStep];
    A(3,3) = 1;
    
    B = ones(3,1);
    C = zeros(1,3);
    C(1)=1;
    
%   Process noise covariance matrix
    R1 = [arEkfInitialisation(5),0,0;...
        0,arEkfInitialisation(6),0;...
        0,0,arEkfInitialisation(7)];

%   Measurement Noise covariance matrix
    R2 = arEkfInitialisation(8);
    
    
    %-------------------------------
    
    
    % Initial values
    P_k_k =  [arEkfInitialisation(9),0,0;...
        0,arEkfInitialisation(10),0;...
        0,0,arEkfInitialisation(11)];
    X_k_k = [rPhi0,rPhi0Star,rFrequency]';
    
end % End of initialisation

% No "input" for this EKF
U = 0;

% Time step consistent with simulation
rTimeStep = arEkfInitialisation(4);

% Define the A matrix as per deliverable 4 report
A(1,:) = [cos(rFrequency*rTimeStep) sin(rFrequency*rTimeStep) 0];
A(2,:) = [-sin(rFrequency*rTimeStep) cos(rFrequency*rTimeStep) 0];
A(3,3) = 1;


% Define the Jacobian as per deliverable 4 report - Note that for very
% small frequencies infinity must be avoided
JA = zeros(3);

if rFrequency<0.001 & rFrequency>=-0.001
    JA(1,:) = [cos(rFrequency*rTimeStep) sin(rFrequency*rTimeStep) rPhi0Star*rTimeStep-rPhi0*rFrequency*rTimeStep^2/2];
    JA(2,:) = [-sin(rFrequency*rTimeStep) cos(rFrequency*rTimeStep) -rPhi0*rTimeStep-rPhi0Star*rFrequency*rTimeStep^2/2];
    JA(3,3) = 1;
else
    JA(1,:) = [cos(rFrequency*rTimeStep) sin(rFrequency*rTimeStep) rPhi0Star*sin(rFrequency*rTimeStep)/rFrequency-rPhi0*(1-cos(rFrequency*rTimeStep))/rFrequency];
    JA(2,:) = [-sin(rFrequency*rTimeStep) cos(rFrequency*rTimeStep) -rPhi0*sin(rFrequency*rTimeStep)/rFrequency-rPhi0Star*(1-cos(rFrequency*rTimeStep))/rFrequency];
    JA(3,3) = 1;
end

% Define B and C Matrices
B = ones(3,1);
C = zeros(1,3);
C(1)=1;

% Kalman Filter
%---------------------------------
% Prediction
X_k1_k = A*X_k_k + B*U;

P_k1_k = JA*P_k_k*JA' + R1;

% Filter
Kf = P_k1_k*C'/(C*P_k1_k*C' + R2);
X_k1_k1 = X_k1_k + Kf*(rEstimatedExcitationForce-C*X_k1_k);
P_k1_k1 = P_k1_k - Kf*(C*P_k1_k*C'+R2)*Kf';


P_k_k = P_k1_k1; % for next cycle;
X_k_k = X_k1_k1; % for next cycle;

rFrequency = X_k_k(3);
rPhi0 = X_k_k(1);
rPhi0Star = X_k_k(2);

rFrequencyOutput = X_k_k(3);
rPhi0Output = X_k_k(1);
rPhi0StarOutput = X_k_k(2);

rAmplitudeOutput = sqrt(rPhi0.^2+rPhi0Star.^2);
